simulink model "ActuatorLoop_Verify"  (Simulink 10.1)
settings: Solver=FixedStepDiscrete  StartTime=0.0  StopTime=10.0  RelTol=1e-3
undefined symbols (not defined in the file or in its folder): Kd, Ki, Kp, sldvsubsys
libraries: sldvlib x1

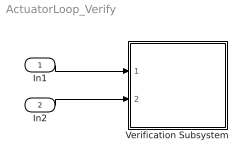
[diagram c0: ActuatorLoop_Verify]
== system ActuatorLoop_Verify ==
  In1 : Inport
  In2 : Inport  Port=2
  Verification Subsystem : Subsystem  Tag=VerificationSubsystem  DisableCoverage=on  LoadFcn=sldvsubsys('check')  TreatAsAtomicUnit=on  SimViewingDevice=on
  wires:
  In1/1 -> Verification Subsystem/1(In1)
  In2/1 -> Verification Subsystem/2(In2)

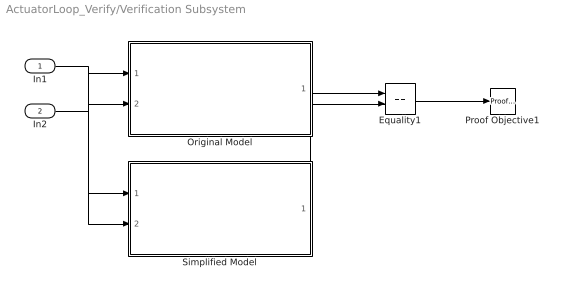
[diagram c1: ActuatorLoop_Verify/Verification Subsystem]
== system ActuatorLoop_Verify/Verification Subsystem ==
  In1 : Inport
  In2 : Inport  Port=2
  Equality1 : RelationalOperator  Operator===  OutDataTypeStr=boolean  RndMeth=Simplest
  Original Model : ModelReference  ModelNameDialog=ActuatorLoop_Original  ParameterArgumentNames=Kd,Ki,Kp  ParameterArgumentValues=[0.00272],[2.73],[0.339]  UsingDefaultArgumentValue=0,0,0  SimulationMode=Normal  ModelReferenceVersion=1.50
  Proof Objective1 : sldvlib/Objectives and Constraints/Proof Objective  enabled=on  customAVTBlockType=Proof Objective  intervals=true  dispValues=on  outEnabled=off  enableStopSim=off
  Simplified Model : ModelReference  ModelNameDialog=ActuatorLoop_New  SimulationMode=Normal  ModelReferenceVersion=1.73
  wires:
  In1/1 -> Original Model/1, Simplified Model/1
  In2/1 -> Original Model/2, Simplified Model/2
  Original Model/1 -> Equality1/1
  Simplified Model/1 -> Equality1/2
  Equality1/1 -> Proof Objective1/1
